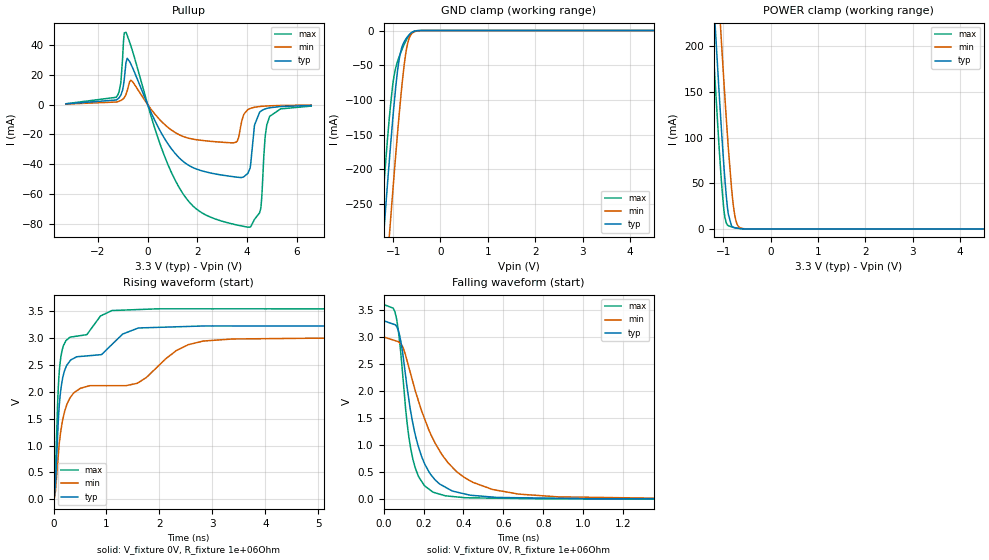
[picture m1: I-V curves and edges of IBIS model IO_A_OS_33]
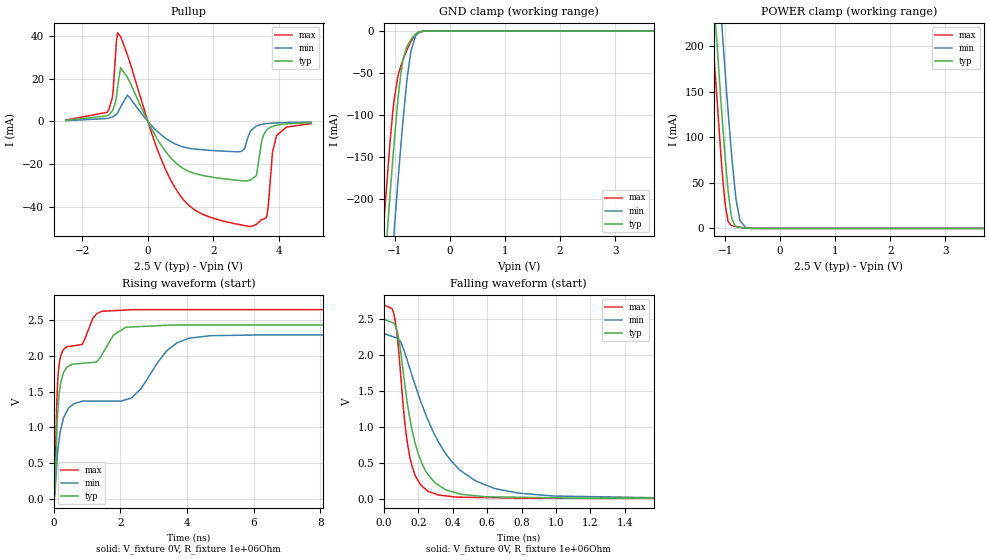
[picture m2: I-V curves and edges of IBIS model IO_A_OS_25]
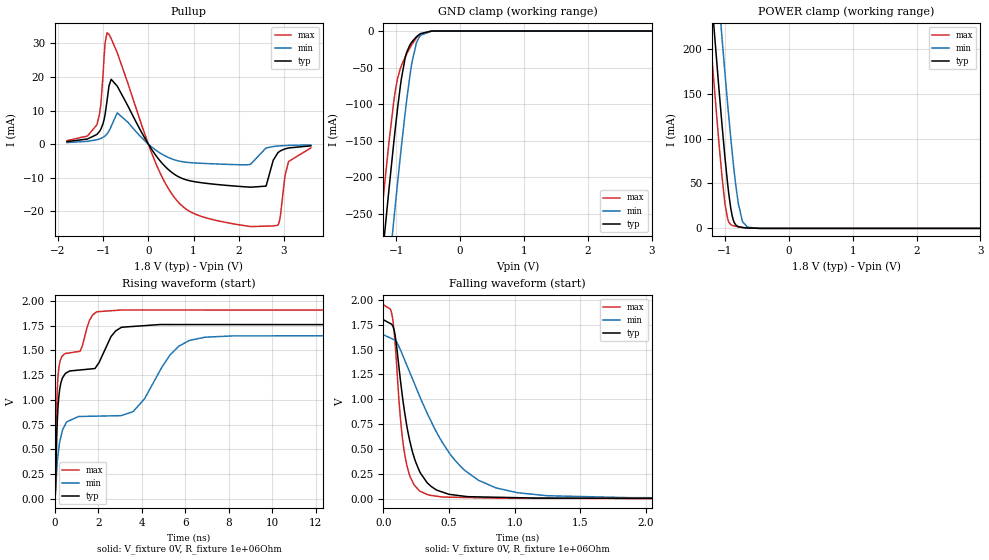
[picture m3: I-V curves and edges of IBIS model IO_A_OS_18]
| Texas Instruments Incorporated
| 4-BIT BIDIRECTIONAL VOLTAGE LEVEL TRANSLATOR FOR OPEN DRAIN APPLICATIONS
| Marketing part#   Voltage Range   Package-type   #pins/pkg drawing
| TXS0104EYZT   1.65V - 5.5V   DSBGA   12-pin YZT
| TXS0104EZGU   1.65V - 5.5V   BGA uStar   12-pin ZXU
| TXS0104EPW   1.65V - 5.5V   TSSOP   14-pin PW
| TXS0104RGY   1.65V - 5.5V   QFN   14-pin RGY
| TXS0104ED   1.65V - 5.5V   SOIC   14-pin D
| This file provides unique models under the [Model Selector] for each Vcc.
| For operation at a specific Vcc, select the appropriate model after each
| [Model Selector] keyword.
[IBIS Ver]   4.1
[Comment char]  |_char
[File Name]   txs0104.ibs
[File Rev]   1.2 | x_die
[Date]   April 24, 2014
[Source]   Model built from spectre simulations at:
   Texas Instruments Incorporated.
   Analog-eLab, HPA
   12500 TI Blvd
   Dallas, TX -75243
   For Support e-mail: elab_ibis@list.ti.com
[Notes]   Revision History
   Rev 1.3  04/24/2014
   - Update package component information
   Rev 1.2: 04/23/2014
   - Update C_comp for IO_A and IO_B Open Source I/O
   Rev 1.1: 04/04/2014
   -Update IO_A_OS and IO_B_OS Open Source I/O buffer models
   -Pullup data is non-monotonic
   Rev 1.0: 04/17/2006
[Disclaimer]  This model is designed as an aid for customers of Texas Instruments
 TI and its licensors and suppliers make no warranties, either expressed
 or implied, with respect to this  model, including the warranties of
 merchantability or fitness for a particular purpose.
 The model is provided solely on an "as is" basis. The entire risk as to
 its quality and performance is with the customer.
[Copyright] (C)Copyright 2014 Texas Instruments Incorporated.
   All rights reserved.
| Component TXS0104E_YZT 12-PIN DSBGA WCSP
[Component]   TXS0104E_YZT
[Manufacturer]   Texas Instruments, Inc.
[Package]   |12 pin DSBGA YZT
|   typ   min   max
R_pkg   0.05   0.05   0.05
L_pkg   0.2n   0.25n   0.2n
C_pkg   0.6p   0.6p   0.6p
[Pin]   signal_name   model_name   R_pin   L_pin   C_pin
A1   B1   IO_A_OS   0.005   0.2nH   0.6pF
B1   B2   IO_A_OS   0.005   0.2nH   0.6pF
C1   B3   IO_A_OS   0.005   0.2nH   0.6pF
D1   B4   IO_A_OS   0.005   0.2nH   0.6pF
A2   VCCB   POWER   0.005   0.2nH   0.6pF
B2   VCCA   POWER   0.005   0.2nH   0.6pF
C2   OE   TXS0104_IN   0.005   0.2nH   0.6pF
D2   GND   GND   0.005   0.2nH   0.6pF
A3   A1   IO_B_OS   0.005   0.2nH   0.6pF
B3   A2   IO_B_OS   0.005   0.2nH   0.6pF
C3   A3   IO_B_OS   0.005   0.2nH   0.6pF
D3   A4   IO_B_OS   0.005   0.2nH   0.6pF
| Component TXS0104E_ZXU 12-PIN BGA uStar Jr
[Component]   TXS0104E_ZXU
[Manufacturer]   Texas Instruments, Inc.
[Package]   |12 pin BGA ZXU
|   typ   min   max
R_pkg   0.0618   0.0506   0.1217
L_pkg   1.1585n   0.8335n   2.9376n
C_pkg   0.1606p   0.1114p   0.2507p
[Pin]   signal_name   model_name   R_pin   L_pin   C_pin
A1   A1   IO_A_OS   0.05305   0.83838n   0.11143p
A2   A2   IO_A_OS   0.05211   1.05760n   0.19326p
A3   A3   IO_A_OS   0.05064   0.88134n   0.13720p
A4   A4   IO_A_OS   0.06387   1.16815n   0.16034p
B1   VCCB   POWER   0.05145   0.83347n   0.15553p
B2   VCCA   POWER   0.12169   2.93757n   0.25068p
B3   OE   TXS0104_IN   0.05176   0.85106n   0.14815p
B4   GND   GND   0.06619   1.25013n   0.15372p
C1   B1   IO_B_OS   0.05242   0.87586n   0.13496p
C2   B2   IO_B_OS   0.05566   1.10959n   0.19262p
C3   B3   IO_B_OS   0.05603   0.87430n   0.13598p
C4   B4   IO_B_OS   0.06667   1.22435n   0.15273p
| Component TXS0104E_PW 14-PIN TSSOP
[Component]   TXS0104E_PW
[Manufacturer]   Texas Instruments, Inc.
[Package]   |14 pin TSSOP PW
|   typ   min   max
R_pkg   3.200e-02   2.900e-02   3.500e-02
L_pkg   2.378e-09   2.170e-09   2.680e-09
C_pkg   3.140e-13   2.700e-13   3.350e-13
[Pin]   signal_name   model_name   R_pin   L_pin   C_pin
1   VCCA   POWER   3.300e-02   2.618e-09   3.300e-13
2   A1   IO_A_OS   3.100e-02   2.313e-09   3.170e-13
3   A2   IO_A_OS   3.000e-02   2.310e-09   3.140e-13
4   A3   IO_A_OS   3.100e-02   2.173e-09   2.720e-13
5   A4   IO_A_OS   3.000e-02   2.204e-09   3.090e-13
6   NC   NC   3.200e-02   2.315e-09   3.170e-13
7   GND   GND   3.500e-02   2.680e-09   3.350e-13
8   OE   TXS0104_IN   3.300e-02   2.640e-09   3.330e-13
9   NC   NC   3.400e-02   2.347e-09   3.190e-13
10   B4   IO_B_OS   2.900e-02   2.277e-09   3.130e-13
11   B3   IO_B_OS   3.100e-02   2.170e-09   2.700e-13
12   B2   IO_B_OS   3.100e-02   2.244e-09   3.110e-13
13   B1   IO_B_OS   3.300e-02   2.343e-09   3.210e-13
14   VCCB   POWER   3.500e-02   2.657e-09   3.320e-13
| Component TXS0104_RGY 14-PIN QFN
[Component]   TXS0104E_RGY
[Manufacturer]   Texas Instruments, Inc.
[Package]   |14 pin QFN RGY
|   typ   min   max
R_pkg   3.300e-02   3.000e-02   3.500e-02
L_pkg   7.380e-10   6.850e-10   7.840e-10
C_pkg   3.160e-13   3.040e-13   3.230e-13
[Pin]   signal_name   model_name   R_pin   L_pin   C_pin
1   VCCA   POWER   3.500e-02   7.840e-10   3.040e-13
2   A1   IO_A_OS   3.400e-02   7.690e-10   3.160e-13
3   A2   IO_A_OS   3.300e-02   7.360e-10   3.210e-13
4   A3   IO_A_OS   3.300e-02   7.390e-10   3.170e-13
5   A4   IO_A_OS   3.100e-02   6.910e-10   3.170e-13
6   NC   NC   3.100e-02   6.970e-10   3.180e-13
7   GND   GND   3.200e-02   7.130e-10   3.160e-13
8   OE   TXS0104_IN   3.500e-02   7.830e-10   3.120e-13
9   NC   NC   3.400e-02   7.680e-10   3.150e-13
10   B4   IO_B_OS   3.400e-02   7.720e-10   3.230e-13
11   B3   IO_B_OS   3.300e-02   7.340e-10   3.170e-13
12   B2   IO_B_OS   3.000e-02   6.880e-10   3.150e-13
13   B1   IO_B_OS   3.000e-02   6.850e-10   3.150e-13
14   VCCB   POWER   3.400e-02   7.730e-10   3.130e-13
| Component TXS0104E_D 14-PIN SOIC
[Component]   TXS0104E_D
[Manufacturer]   Texas Instruments, Inc.
[Package]   |14 pin SOIC D
|   typ   min   max
R_pkg   3.100e-02   2.800e-02   3.400e-02
L_pkg   3.109e-09   2.462e-09   3.889e-09
C_pkg   4.730e-13   3.630e-13   6.280e-13
[Pin]   signal_name   model_name   R_pin   L_pin   C_pin
1   VCCA   POWER   3.300e-02   3.854e-09   6.220e-13
2   A1   IO_A_OS   3.200e-02   3.188e-09   4.730e-13
3   A2   IO_A_OS   2.800e-02   2.462e-09   3.770e-13
4   A3   IO_A_OS   3.100e-02   2.596e-09   3.630e-13
5   A4   IO_A_OS   2.800e-02   2.521e-09   3.720e-13
6   NC   NC   3.400e-02   3.250e-09   4.760e-13
7   GND   GND   3.400e-02   3.889e-09   6.280e-13
8   OE   TXS0104_IN   3.400e-02   3.889e-09   6.280e-13
9   NC   NC   3.400e-02   3.250e-09   4.760e-13
10   B4   IO_B_OS   2.800e-02   2.521e-09   3.720e-13
11   B3   IO_B_OS   3.100e-02   2.596e-09   3.640e-13
12   B2   IO_B_OS   2.800e-02   2.462e-09   3.770e-13
13   B1   IO_B_OS   3.200e-02   3.188e-09   4.730e-13
14   VCCB   POWER   3.300e-02   3.854e-09   6.220e-13
| Model IO_A_OS
[Model Selector]   IO_A_OS
IO_A_OS_18   1.8 volt VCCA, Open_Source I/O
IO_A_OS_25   2.5 volt VCCA, Open_Source I/O
IO_A_OS_33   3.3 volt VCCA, Open_Source I/O
| Model IO_B_OS
[Model Selector]   IO_B_OS
IO_B_OS_25   2.5 volt VCCB, Open_Source I/O
IO_B_OS_33   3.3 volt VCCB, Open_Source I/O
IO_B_OS_50   5 volt VCCB, Open_Source I/O
| Model TXS0104_IN
[Model Selector]   TXS0104_IN
TXS0104_IN_18   1.8 volt Vcc
TXS0104_IN_25   2.5 volt Vcc
TXS0104_IN_33   3.3 volt Vcc
TXS0104_IN_50   5 volt Vcc
| Models and submodels in the file (10): IO_A_OS_33 (I/O_open_source), IO_A_OS_25 (I/O_open_source), IO_A_OS_18 (I/O_open_source), IO_B_OS_50 (I/O_open_source), IO_B_OS_33 (I/O_open_source), IO_B_OS_25 (I/O_open_source), TXS0104_IN_18 (Input), TXS0104_IN_25 (Input), TXS0104_IN_33 (Input), TXS0104_IN_50 (Input)
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[Model]   IO_A_OS_33
Model_type   I/O_open_source
Polarity   Non-Inverting
Vinl=0.8
Vinh=2.0
Vmeas = 1.65
Vref = 0
Cref = 15pF
Rref = 1000000
|   typ   min   max
C_comp   4.179pF   4.145pF   4.223pF
[Voltage Range]   3.3   3   3.6
[Temperature Range]   27   125   -40
[Pullup Reference]   3.3   3   3.6
[Pulldown Reference]   0   0   0
[Power Clamp Reference]   3.3   3   3.6
[GND Clamp Reference]   0   0   0
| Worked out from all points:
|   slope of the pullup table from 0 to 0.495 V, typ, clamps not added: 28.3 ohm
|   GND clamp passes 1 mA (typ) near -0.55 V on its own axis
|   POWER clamp passes 1 mA (typ) near -0.73 V on its own axis
|   falling waveform, V_fixture 0V, R_fixture 1e+06Ohm: 20-80 % time 107ps typ, 213ps min, 67.1ps max; typ from 3.3 V to 0 V
|   rising waveform, V_fixture 0V, R_fixture 1e+06Ohm: 20-80 % time 359ps typ, 1.82ns min, 154ps max; typ from 0 V to 3.3 V
[GND Clamp]
|   Voltage   I(typ)   I(min)   I(max)
-3.3V     -2.336A    -2.441A    -2.271A
-1.3V     -385.4mA   -497.2mA   -316.4mA
-1.251V   -339.6mA   -451.2mA   -271.1mA
-1.231V   -321.5mA   -432.9mA   -253.2mA
-1.122V   -223.6mA   -333.4mA   -158.8mA
-1.073V   -180.8mA   -289mA     -120mA
-983.4mV  -108.9mA   -211.3mA   -66.6mA
-864.6mV  -38.22mA   -115.1mA   -36.31mA
-785.4mV  -18.96mA   -60.6mA    -22.93mA
-716.1mV  -10.71mA   -26.1mA    -13.09mA
-577.5mV  -1.747mA   -2.785mA   -1.605mA
6.59V     0A         0A         0A
[Pullup]
|   Voltage   I(typ)   I(min)   I(max)
-3.3V     446.4uA    328.2uA    543.5uA
-1.261V   3.163mA    1.737mA    5.075mA
-874.5mV  28.15mA    6.783mA    48.48mA
-656.7mV  26.45mA    16.1mA     38.31mA
1.363V    -37.2mA    -20.97mA   -58.3mA
3.561V    -48.63mA   -25.21mA   -80.67mA
4.036V    -46.17mA   -3.435mA   -82.27mA
4.303V    -13.87mA   -1.814mA   -77.05mA
4.551V    -4.568mA   -1.245mA   -70.25mA
4.729V    -2.973mA   -1.013mA   -22.54mA
4.907V    -2.187mA   -852.1uA   -8.212mA
6.59V     -610.1uA   -337.5uA   -1.006mA
[POWER Clamp]
|   Voltage   I(typ)   I(min)   I(max)
-3.3V     2.291A     2.383A     2.236A
-1.261V   304.2mA    404.1mA    241.9mA
-1.221V   267.9mA    367.8mA    205.7mA
-1.181V   232.1mA    331.7mA    170mA
-1.073V   137mA      234.7mA    77.56mA
-1.043V   112.5mA    209mA      55.19mA
-973.5mV  59.96mA    151mA      15.7mA
-894.3mV  16.56mA    89.79mA    3.583mA
-825mV    3.303mA    44.77mA    2.229mA
-765.6mV  1.354mA    17.89mA    1.511mA
-617.1mV  302.9uA    757.1uA    311.9uA
6.59V     0A         0A         0A
[Ramp]
R_load = 1e+06
|   typ   min   max
dV/dt_r   1.97995/3.46931e-10   1.79694/1.82562e-09   2.15996/1.51255e-10
dV/dt_f   1.97995/1.07308e-10   1.79992/2.1221e-10   2.15996/6.70113e-11
[Falling Waveform]
V_fixture = 0V
V_fixture_min = 0V
V_fixture_max = 0V
R_fixture = 1e+06Ohm
C_fixture = 0F
|   Time   V(typ)   V(min)   V(max)
0s        3.3V       3V         3.6V
63.1ps    3.204V     2.925V     3.365V
86.51ps   2.911V     2.867V     2.678V
125.3ps   1.87V      2.454V     1.182V
171ps     1.012V     1.859V     455.4mV
256.5ps   365.4mV    1.05V      121.9mV
407.2ps   98.8mV     398.6mV    30.14mV
676.9ps   29.62mV    96.81mV    15.36mV
1.467ns   8.948mV    15.64mV    4.843mV
19.9ns    0V         0V         0V
[Rising Waveform]
V_fixture = 0V
V_fixture_min = 0V
V_fixture_max = 0V
R_fixture = 1e+06Ohm
C_fixture = 0F
|   Time   V(typ)   V(min)   V(max)
0s        0V         4.976mV    0V
28.86ps   199.6mV    101.2mV    337.6mV
101.2ps   1.648V     958.7mV    2.282V
179.3ps   2.287V     1.507V     2.837V
506.3ps   2.659V     2.066V     3.046V
1.103ns   2.881V     2.115V     3.513V
1.607ns   3.189V     2.176V     3.532V
2.55ns    3.217V     2.879V     3.545V
3.385ns   3.227V     2.984V     3.545V
19.9ns    3.3V       3V         3.6V
[Model]   IO_A_OS_25
Model_type   I/O_open_source
Polarity   Non-Inverting
Vinl=0.7
Vinh=1.7
Vmeas = 1.25
Vref = 0
Cref = 15pF
Rref = 1000000
|   typ   min   max
C_comp   4.179pF   4.145pF   4.223pF
[Voltage Range]   2.5   2.3   2.7
[Temperature Range]   27   125   -40
[Pullup Reference]   2.5   2.3   2.7
[Pulldown Reference]   0   0   0
[Power Clamp Reference]   2.5   2.3   2.7
[GND Clamp Reference]   0   0   0
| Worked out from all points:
|   slope of the pullup table from 0 to 0.375 V, typ, clamps not added: 36.2 ohm
|   GND clamp passes 1 mA (typ) near -0.55 V on its own axis
|   POWER clamp passes 1 mA (typ) near -0.73 V on its own axis
|   falling waveform, V_fixture 0V, R_fixture 1e+06Ohm: 20-80 % time 119ps typ, 270ps min, 73ps max; typ from 2.5 V to 0 V
|   rising waveform, V_fixture 0V, R_fixture 1e+06Ohm: 20-80 % time 1.36ns typ, 2.94ns min, 765ps max; typ from 0 V to 2.5 V
[GND Clamp]
|   Voltage   I(typ)   I(min)   I(max)
-2.5V     -1.547A    -1.655A    -1.48A
-1.225V   -316.1mA   -427.4mA   -247.9mA
-1.097V   -202.2mA   -311.3mA   -139.1mA
-1.015V   -133.3mA   -238.5mA   -82.05mA
-947.5mV  -83.17mA   -181.1mA   -54.24mA
-895mV    -51.71mA   -138.5mA   -42.1mA
-850mV    -33.13mA   -104.2mA   -33.69mA
-775mV    -17.47mA   -54.45mA   -21.33mA
-707.5mV  -9.886mA   -23.02mA   -12.02mA
-625mV    -3.786mA   -6.106mA   -4.042mA
-572.5mV  -1.592mA   -2.56mA    -1.436mA
4.992V    0A         0A         0A
[Pullup]
|   Voltage   I(typ)   I(min)   I(max)
-2.5V     548.7uA    380.4uA    701uA
-1.195V   3.139mA    1.582mA    5.563mA
-1.067V   5.464mA    2.246mA    13.55mA
-925mV    15.98mA    4.005mA    41.63mA
-835mV    25.28mA    6.811mA    39.87mA
950mV     -20.67mA   -11.29mA   -33.96mA
2.84V     -27.78mA   -14.1mA    -48.52mA
3.147V    -27.36mA   -4.279mA   -49.34mA
3.643V    -3.813mA   -970.7uA   -43.86mA
3.808V    -2.29mA    -758.7uA   -14.5mA
3.935V    -1.733mA   -648.1uA   -6.546mA
4.992V    -559.4uA   -290.4uA   -1.002mA
[POWER Clamp]
|   Voltage   I(typ)   I(min)   I(max)
-2.5V     1.502A     1.596A     1.445A
-1.24V    285.3mA    385.2mA    223mA
-1.218V   264.7mA    364.6mA    202.5mA
-1.067V   132.8mA    230.4mA    73.66mA
-1.052V   120.4mA    217.4mA    62.27mA
-992.5mV  73.5mA     166.6mA    23.96mA
-947.5mV  42.97mA    130.1mA    8.442mA
-880mV    11.97mA    79.65mA    3.172mA
-797.5mV  2.026mA    30.63mA    1.877mA
-730mV    961.2uA    8.682mA    1.146mA
-617.5mV  304.4uA    762.7uA    313.8uA
4.992V    0A         0A         0A
[Ramp]
R_load = 1e+06
|   typ   min   max
dV/dt_r   1.49995/1.35743e-09   1.37745/2.93411e-09   1.61997/7.90657e-10
dV/dt_f   1.49995/1.19159e-10   1.37992/2.68834e-10   1.61997/7.28035e-11
[Falling Waveform]
V_fixture = 0V
V_fixture_min = 0V
V_fixture_max = 0V
R_fixture = 1e+06Ohm
C_fixture = 0F
|   Time   V(typ)   V(min)   V(max)
0s        2.5V       2.3V       2.7V
62.56ps   2.427V     2.25V      2.519V
86.42ps   2.223V     2.216V     2.038V
128ps     1.469V     1.983V     922.1mV
177.3ps   812.8mV    1.613V     351.8mV
250.4ps   354.9mV    1.129V     115mV
420.1ps   80.88mV    452.2mV    22.65mV
784ps     19.79mV    76.82mV    8.199mV
1.606ns   6.223mV    12.28mV    3.39mV
19.9ns    0V         0V         0V
[Rising Waveform]
V_fixture = 0V
V_fixture_min = 0V
V_fixture_max = 0V
R_fixture = 1e+06Ohm
C_fixture = 0F
|   Time   V(typ)   V(min)   V(max)
0s        0V         4.118mV    0V
29.26ps   128.1mV    63.7mV     218.8mV
106.5ps   1.119V     602.5mV    1.563V
205.2ps   1.618V     963mV      2.001V
623.2ps   1.889V     1.337V     2.147V
1.431ns   2.011V     1.369V     2.627V
2.154ns   2.404V     1.387V     2.646V
3.686ns   2.436V     2.184V     2.651V
4.707ns   2.436V     2.286V     2.651V
19.9ns    2.5V       2.3V       2.7V
[Model]   IO_A_OS_18
Model_type   I/O_open_source
Polarity   Non-Inverting
Vinl=0.5775
Vinh=1.2675
Vmeas = 0.9
Vref = 0
Cref = 15pF
Rref = 1000000
|   typ   min   max
C_comp   4.179pF   4.145pF   4.223pF
[Voltage Range]   1.8   1.65   1.95
[Temperature Range]   27   125   -40
[Pullup Reference]   1.8   1.65   1.95
[Pulldown Reference]   0   0   0
[Power Clamp Reference]   1.8   1.65   1.95
[GND Clamp Reference]   0   0   0
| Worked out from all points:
|   slope of the pullup table from 0 to 0.27 V, typ, clamps not added: 52.4 ohm
|   GND clamp passes 1 mA (typ) near -0.49 V on its own axis
|   POWER clamp passes 1 mA (typ) near -0.73 V on its own axis
|   falling waveform, V_fixture 0V, R_fixture 1e+06Ohm: 20-80 % time 140ps typ, 400ps min, 80.6ps max; typ from 1.8 V to 0 V
|   rising waveform, V_fixture 0V, R_fixture 1e+06Ohm: 20-80 % time 2.11ns typ, 4.8ns min, 1.23ns max; typ from 0 V to 1.8 V
[GND Clamp]
|   Voltage   I(typ)   I(min)   I(max)
-1.8V     -862.6mA   -973.2mA   -794mA
-1.255V   -343.2mA   -454.8mA   -274.6mA
-1.174V   -269.4mA   -380.2mA   -202.5mA
-1.039V   -152.4mA   -259.1mA   -96.32mA
-979.2mV  -105.7mA   -207.7mA   -64.88mA
-919.8mV  -65.45mA   -158.4mA   -47.32mA
-860.4mV  -36.66mA   -111.9mA   -35.55mA
-752.4mV  -14.6mA    -42.17mA   -17.99mA
-682.2mV  -7.675mA   -15.57mA   -9.107mA
-622.8mV  -3.668mA   -5.888mA   -3.893mA
-385.2mV  -15.02uA   -57.54uA   -4.741uA
3.595V    0A         0A         0A
[Pullup]
|   Voltage   I(typ)   I(min)   I(max)
-1.8V     744.4uA    464.9uA    1.038mA
-1.141V   2.859mA    1.302mA    5.723mA
-1.055V   4.342mA    1.683mA    11.46mA
-914.4mV  12.86mA    3.03mA     33.17mA
-822.6mV  19.33mA    5.282mA    31.45mA
-687.6mV  17.28mA    9.323mA    27.22mA
230.4mV   -4.505mA   -2.395mA   -7.724mA
910.8mV   -10.89mA   -5.491mA   -20.02mA
2.601V    -12.51mA   -1.175mA   -24.43mA
2.866V    -2.572mA   -559.2uA   -24.13mA
3.103V    -1.138mA   -373.7uA   -5.16mA
3.595V    -507.5uA   -219.5uA   -1.142mA
[POWER Clamp]
|   Voltage   I(typ)   I(min)   I(max)
-1.8V     817.9mA    915.4mA    758.1mA
-1.238V   283.8mA    383.7mA    221.5mA
-1.179V   229.9mA    329.5mA    167.9mA
-1.049V   117.9mA    214.7mA    59.98mA
-995.4mV  75.64mA    169mA      25.43mA
-957.6mV  49.33mA    138.1mA    10.71mA
-909mV    22.47mA    100.6mA    4.21mA
-860.4mV  7.457mA    66.39mA    2.769mA
-790.2mV  1.824mA    27.35mA    1.79mA
-725.4mV  922.2uA    7.848mA    1.102mA
-644.4mV  419.6uA    1.294mA    463.4uA
3.595V    0A         0A         0A
[Ramp]
R_load = 1e+06
|   typ   min   max
dV/dt_r   1.07995/2.10199e-09   0.987597/4.79622e-09   1.16997/1.2352e-09
dV/dt_f   1.07995/1.39608e-10   0.989916/4.00019e-10   1.16997/8.03308e-11
[Falling Waveform]
V_fixture = 0V
V_fixture_min = 0V
V_fixture_max = 0V
R_fixture = 1e+06Ohm
C_fixture = 0F
|   Time   V(typ)   V(min)   V(max)
0s        1.8V       1.65V      1.95V
69.23ps   1.741V     1.607V     1.819V
138.2ps   1.095V     1.47V      685.7mV
193.6ps   624.7mV    1.293V     257.9mV
283.7ps   253.8mV    1.006V     71.77mV
446.6ps   67.89mV    571.9mV    17.04mV
622.1ps   23.55mV    282.1mV    12.03mV
864.6ps   14.39mV    106.7mV    5.496mV
1.868ns   4.17mV     10.68mV    1.744mV
19.9ns    0V         0V         0V
[Rising Waveform]
V_fixture = 0V
V_fixture_min = 0V
V_fixture_max = 0V
R_fixture = 1e+06Ohm
C_fixture = 0F
|   Time   V(typ)   V(min)   V(max)
0s        0V         3.866mV    0V
27.97ps   81.24mV    41.07mV    142.9mV
108.8ps   747.6mV    354.1mV    1.065V
229.7ps   1.112V     574.3mV    1.379V
1.158ns   1.302V     831.6mV    1.491V
1.921ns   1.34V      834.9mV    1.889V
3.077ns   1.734V     841.7mV    1.909V
5.698ns   1.761V     1.542V     1.908V
6.9ns     1.761V     1.633V     1.908V
19.9ns    1.8V       1.65V      1.95V
